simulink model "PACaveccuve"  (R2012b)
settings: Solver=ode45  StartTime=0.0  StopTime=6000  RelTol=1e-3
libraries: fl_lib x9, nesl_utility x6

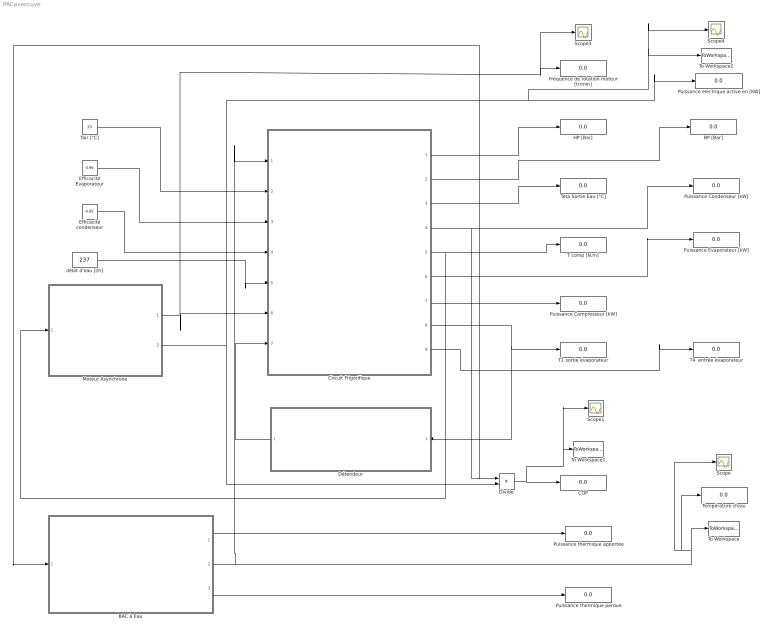
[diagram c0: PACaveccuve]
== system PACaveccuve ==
  BAC à Eau : Subsystem
  BP [Bar] : Display
  COP : Display
  Circuit Frigorifique : Subsystem
  Divide : Product  Inputs=*/
  Détendeur : Subsystem
  Efficacité Evaporateur : Constant  Value=0.99
  Efficacité condenseur : Constant  Value=0.95
  Fréquence de rotation moteur [tr/min] : Display
  HP [Bar] : Display
  Moteur Asynchrone : Subsystem
  Puissance Compresseur [kW] : Display
  Puissance Condenseur [kW] : Display
  Puissance Evaporateur [kW] : Display
  Puissance electrique active en [KW] : Display
  Puissance thermique apportée : Display
  Puissance thermique perdue : Display
  Scope{,1,3..4} (4 alike) : Scope
  T comp [N.m] : Display
  T1 sortie évaporateur : Display
  T4  entrée évaporateur : Display
  Tair [°C] : Constant  Value=23
  Température d'eau : Display
  Teta Sortie Eau [°C] : Display
  To Workspace : ToWorkspace  VariableName=Ts  SampleTime=-1  SaveFormat=Timeseries
  To Workspace1 : ToWorkspace  VariableName=COP  SampleTime=-1  SaveFormat=Timeseries
  To Workspace2 : ToWorkspace  VariableName=Pelec  SampleTime=-1  SaveFormat=Timeseries
  débit d'eau [l/h] : Constant  Value=237
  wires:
  Efficacité Evaporateur/1 -> Circuit Frigorifique/3(Eff Evapo)
  débit d'eau [l/h]/1 -> Circuit Frigorifique/5(Qv eau [l/h])
  Circuit Frigorifique/1(HP [bar]) -> HP [Bar]/1
  Circuit Frigorifique/2(BP [bar]) -> BP [Bar]/1
  Circuit Frigorifique/3(Tse [°C]) -> Teta Sortie Eau [°C]/1
  Circuit Frigorifique/5(Tm [N.m]) -> Moteur Asynchrone/1(Tm [N.m]), T comp [N.m]/1
  Circuit Frigorifique/9(T4 [°C]) -> T4  entrée évaporateur/1
  Circuit Frigorifique/8(T1 [°C]) -> Détendeur/1(T1), T1 sortie évaporateur/1
  Circuit Frigorifique/6(Pevapo [kW]) -> Puissance Evaporateur [kW]/1
  Divide/1 -> To Workspace1/1, Scope1/1, COP/1
  Circuit Frigorifique/7(Pcomp [kW]) -> Puissance Compresseur [kW]/1
  Efficacité condenseur/1 -> Circuit Frigorifique/4(effc)
  Détendeur/1(BP [Bar]) -> Circuit Frigorifique/7(BP[Bar])
  Moteur Asynchrone/2(Puissance Electrique active [W]) -> Scope4/1, To Workspace2/1, Puissance electrique active en [KW]/1, Divide/2
  Moteur Asynchrone/1(N [tr/min]) -> Scope3/1, Fréquence de rotation moteur [tr/min]/1, Circuit Frigorifique/6(N [tr/min])
  Tair [°C]/1 -> Circuit Frigorifique/2(Tair [°C])
  Circuit Frigorifique/4(Pcond [kW]) -> BAC à Eau/1(" Puissance Condenseur [kW]"), Divide/1, Puissance Condenseur [kW]/1
  BAC à Eau/2(Température du BAC [°C]) -> Scope/1, Température d'eau/1, To Workspace/1, Circuit Frigorifique/1(Tee [°C])
  BAC à Eau/1(Puissance Condenseur [W]) -> Puissance thermique apportée/1
  BAC à Eau/3(Puissance thermique perdue [W]) -> Puissance thermique perdue/1

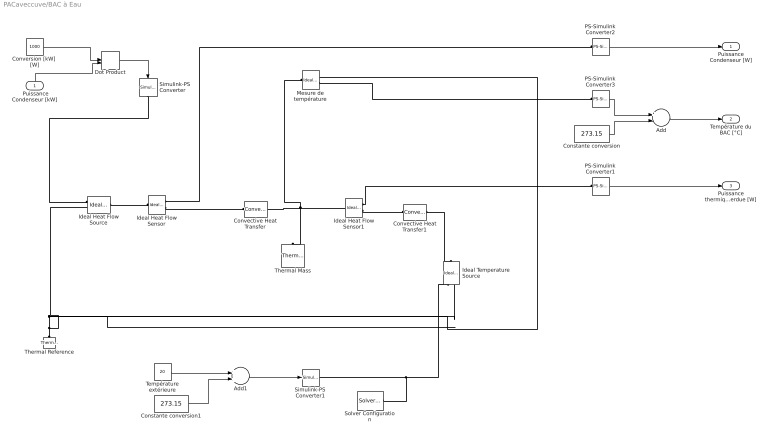
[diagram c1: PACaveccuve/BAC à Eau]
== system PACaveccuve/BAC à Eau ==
  " Puissance Condenseur [kW]" : Inport
  Add : Sum  Inputs=+-
  Add1 : Sum
  Constante conversion : Constant  Value=273.15
  Constante conversion1 : Constant  Value=273.15
  Convective Heat Transfer : fl_lib/Thermal/Thermal Elements/Convective Heat Transfer  area=1 m^2  heat_tr_coeff=1000000 W/(m^2 * K)  Q_Log=off  T_Log=off  LocalVarNames=|Q|T  LocalVarDescs=|Q|T  LocalVarLogging=[0 0]
  Convective Heat Transfer1 : fl_lib/Thermal/Thermal Elements/Convective Heat Transfer  area=1 m^2  heat_tr_coeff=10.3 W/(m^2 * K)  Q_Log=off  T_Log=off  LocalVarNames=|Q|T  LocalVarDescs=|Q|T  LocalVarLogging=[0 0]
  Conversion [kW]  [W] : Constant  Value=1000
  Dot Product : DotProduct
  Ideal Heat Flow Sensor : fl_lib/Thermal/Thermal Sensors/Ideal Heat Flow Sensor  Q_Log=off  T_Log=off  LocalVarNames=|Q|T  LocalVarDescs=|Q|T  LocalVarLogging=[0 0]
  Ideal Heat Flow Sensor1 : fl_lib/Thermal/Thermal Sensors/Ideal Heat Flow Sensor  Q_Log=off  T_Log=off  LocalVarNames=|Q|T  LocalVarDescs=|Q|T  LocalVarLogging=[0 0]
  Ideal Heat Flow Source : fl_lib/Thermal/Thermal Sources/Ideal Heat Flow Source  Q_Log=off  T_Log=off  LocalVarNames=|Q|T  LocalVarDescs=|Q|T  LocalVarLogging=[0 0]
  Ideal Temperature Source : fl_lib/Thermal/Thermal Sources/Ideal Temperature Source  Q_Log=off  T_Log=off  LocalVarNames=|Q|T  LocalVarDescs=|Q|T  LocalVarLogging=[0 0]
  Mesure de température : fl_lib/Thermal/Thermal Sensors/Ideal Temperature Sensor  Qs_Log=off  Ts_Log=off  LocalVarNames=|Qs|Ts  LocalVarDescs=|Qs|Ts  LocalVarLogging=[]
  PS-Simulink Converter1 : nesl_utility/PS-Simulink Converter  PhysicalDomain=network_engine_domain  LeftPortType=input  RightPortType=output  SubClassName=ps_output  PseudoPeriodic=off  Frequencies=[]  Unit=1  AffineConversion=off
  PS-Simulink Converter2 : nesl_utility/PS-Simulink Converter  PhysicalDomain=network_engine_domain  LeftPortType=input  RightPortType=output  SubClassName=ps_output  PseudoPeriodic=off  Frequencies=[]  Unit=1  AffineConversion=off
  PS-Simulink Converter3 : nesl_utility/PS-Simulink Converter  PhysicalDomain=network_engine_domain  LeftPortType=input  RightPortType=output  SubClassName=ps_output  PseudoPeriodic=off  Frequencies=[]  Unit=1  AffineConversion=off
  Simulink-PS Converter : nesl_utility/Simulink-PS Converter  PhysicalDomain=network_engine_domain  LeftPortType=input  RightPortType=output  SubClassName=ps_input  PseudoPeriodic=off  Frequencies=[]  NoiseDistribution=none  NoiseParameters=[]  Unit=1  AffineConversion=off  InputFilterTimeConstant=.001  UdotUserProvided=1  SimscapeFilterOrder=1  InputFiltering=off
  Simulink-PS Converter1 : nesl_utility/Simulink-PS Converter  PhysicalDomain=network_engine_domain  LeftPortType=input  RightPortType=output  SubClassName=ps_input  PseudoPeriodic=off  Frequencies=[]  NoiseDistribution=none  NoiseParameters=[]  Unit=K  AffineConversion=on  InputFilterTimeConstant=.001  UdotUserProvided=1  SimscapeFilterOrder=1  InputFiltering=off
  Solver Configuration : nesl_utility/Solver Configuration  PhysicalDomain=network_engine_domain  LeftPortType=input  RightPortType=generic  SubClassName=solver  Accelerate=off  Profile=off  UseLocalSampling=off  FrequencyDomain=off  Tones=[]  Harmonics=[]  UseCCode=off  SimulateNoise=off  EnableSwitchedLinearOptims=on  DoDC=off  ResidualTolerance=1e-9  UseLocalSolver=off  LocalSolverChoice=NE_BACKWARD_EULER_ADVANCER  LocalSolverSampleTime=.001  DoFixedCost=off  MaxNonlinIter=3  MaxModeIter=2  LinearAlgebra=Sparse  DelaysMemoryBudget=1024
  Température extérieure : Constant  Value=20
  Thermal Mass : fl_lib/Thermal/Thermal Elements/Thermal Mass  mass=19.9 kg  sp_heat=4185 J/kg/K  init_temp=23.25 C  Q_Log=off  LocalVarNames=|Q  LocalVarDescs=|Q  LocalVarLogging=0
  Thermal Reference : fl_lib/Thermal/Thermal Elements/Thermal Reference  Q_Log=off  LocalVarNames=|Q  LocalVarDescs=|Q  LocalVarLogging=0
  Puissance Condenseur [W] : Outport
  Température du BAC [°C] : Outport  Port=2
  Puissance thermique perdue [W] : Outport  Port=3
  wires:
  " Puissance Condenseur [kW]"/1 -> Dot Product/2
  PS-Simulink Converter3/1 -> Add/1
  Add/1 -> Température du BAC [°C]/1
  Constante conversion/1 -> Add/2
  Dot Product/1 -> Simulink-PS Converter/1
  Conversion [kW]  [W]/1 -> Dot Product/1
  PS-Simulink Converter1/1 -> Puissance thermique perdue [W]/1
  PS-Simulink Converter2/1 -> Puissance Condenseur [W]/1
  Add1/1 -> Simulink-PS Converter1/1
  Température extérieure/1 -> Add1/1
  Constante conversion1/1 -> Add1/2
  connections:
  Thermal Reference/LConn1 -- Ideal Temperature Source/RConn2 -- Mesure de température/RConn1 -- Ideal Heat Flow Source/RConn2
  Mesure de température/LConn1 -- Thermal Mass/LConn1 -- Ideal Heat Flow Sensor1/LConn1 -- Convective Heat Transfer/RConn1
  Solver Configuration/RConn1 -- Ideal Temperature Source/RConn1 -- Simulink-PS Converter1/RConn1
  Simulink-PS Converter/RConn1 -- Ideal Heat Flow Source/RConn1
  Convective Heat Transfer1/RConn1 -- Ideal Temperature Source/LConn1
  PS-Simulink Converter3/LConn1 -- Mesure de température/RConn2
  Ideal Heat Flow Source/LConn1 -- Ideal Heat Flow Sensor/LConn1
  Ideal Heat Flow Sensor/RConn2 -- Convective Heat Transfer/LConn1
  Ideal Heat Flow Sensor1/RConn2 -- Convective Heat Transfer1/LConn1
  Ideal Heat Flow Sensor1/RConn1 -- PS-Simulink Converter1/LConn1
  Ideal Heat Flow Sensor/RConn1 -- PS-Simulink Converter2/LConn1

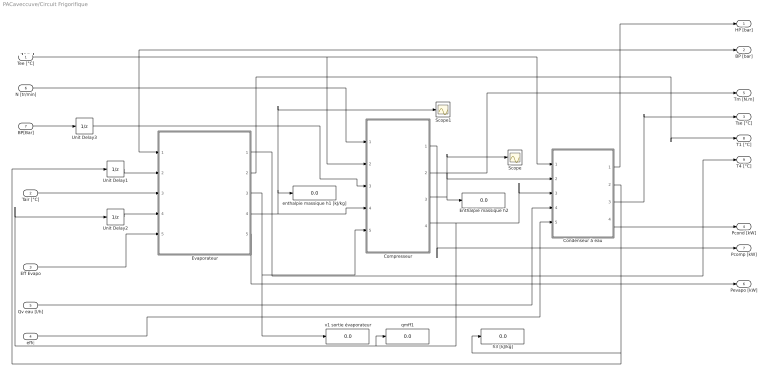
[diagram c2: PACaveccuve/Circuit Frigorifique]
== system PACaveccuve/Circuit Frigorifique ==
  note: +++++
  Tee [°C] : Inport
  Tair [°C] : Inport  Port=2
  Eff Evapo : Inport  Port=3
  effc : Inport  Port=4
  Qv eau [l/h] : Inport  Port=5
  N [tr/min] : Inport  Port=6
  BP[Bar] : Inport  Port=7
  Compresseur : Subsystem
  Condenseur à eau : Subsystem
  Enthalpie massique h2 : Display
  Evaporateur : Subsystem
  Scope : Scope
  Scope1 : Scope
  Unit Delay1 : UnitDelay  InitialCondition=300  SampleTime=-1
  Unit Delay2 : UnitDelay  InitialCondition=0.00001  SampleTime=-1
  Unit Delay3 : UnitDelay  InitialCondition=2.5  SampleTime=-1
  enthalpie massique h1 [kJ/kg] : Display
  h3 [kJ/kg] : Display
  qmff1 : Display
  v1 sortie évaporateur : Display
  HP [bar] : Outport
  BP [bar] : Outport  Port=2
  Tse [°C] : Outport  Port=3
  Pcond [kW] : Outport  Port=4
  Tm [N.m] : Outport  Port=5
  Pevapo [kW] : Outport  Port=6
  Pcomp [kW] : Outport  Port=7
  T1 [°C] : Outport  Port=8
  T4 [°C] : Outport  Port=9
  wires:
  Evaporateur/2(T1 [°C]) -> T1 [°C]/1
  N [tr/min]/1 -> Compresseur/1(N [tr/min])
  Evaporateur/5(Pévapo [kW]) -> Pevapo [kW]/1
  Tair [°C]/1 -> Evaporateur/3(Tair [°C])
  Condenseur à eau/3(Tse [°C]) -> Tse [°C]/1
  Unit Delay2/1 -> Evaporateur/4(qmff [kg/s])
  Condenseur à eau/1(HP [bar]) -> HP [bar]/1
  BP[Bar]/1 -> Unit Delay3/1
  Compresseur/4(qmff [kg/s]) -> Unit Delay2/1, qmff1/1, Condenseur à eau/3(qmff [kg/s])
  Tee [°C]/1 -> Compresseur/2(Tee [°C]), Condenseur à eau/1(Tee [°C])
  Eff Evapo/1 -> Evaporateur/5(Eff)
  Qv eau [l/h]/1 -> Condenseur à eau/4(qveau [l/h])
  Evaporateur/3(v1 [m3/kg]) -> v1 sortie évaporateur/1, Compresseur/5(v1 [m3/kg])
  Condenseur à eau/2(h3 [kJ/kg]) -> Unit Delay1/1, h3 [kJ/kg]/1
  Evaporateur/4(h1 [kJ/kg]) -> Compresseur/4(h1 [kJ/kg]), Scope1/1, enthalpie massique h1 [kJ/kg]/1
  Compresseur/3(h2 [kJ/kg]) -> Scope/1, Condenseur à eau/2(h2 [kJ/kg]), Enthalpie massique h2/1
  Compresseur/2(Tm [N.m]) -> Tm [N.m]/1
  Evaporateur/1(T4 [°C]) -> T4 [°C]/1
  Condenseur à eau/4(Pcond [kW]) -> Pcond [kW]/1
  Unit Delay1/1 -> Evaporateur/2(h3 [kJ/kg])
  Compresseur/1(Pcomp [kW]) -> Pcomp [kW]/1
  effc/1 -> Condenseur à eau/5(effc)
  Unit Delay3/1 -> BP [bar]/1, Compresseur/3(BP [bar]), Evaporateur/1(BP [bar])

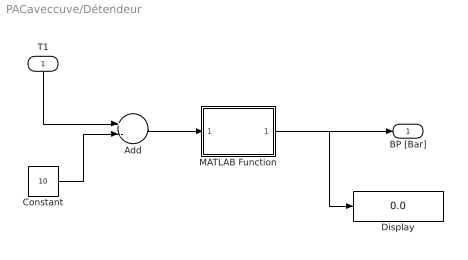
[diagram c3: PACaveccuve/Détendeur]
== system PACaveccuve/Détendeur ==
  T1 : Inport
  Add : Sum  Inputs=+-
  Constant : Constant  Value=10
  Display : Display
  MATLAB Function : MATLAB Function  TreatAsAtomicUnit=on
  BP [Bar] : Outport
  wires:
  Add/1 -> MATLAB Function/1(T)
  T1/1 -> Add/1
  Constant/1 -> Add/2
  MATLAB Function/1(BP) -> Display/1, BP [Bar]/1

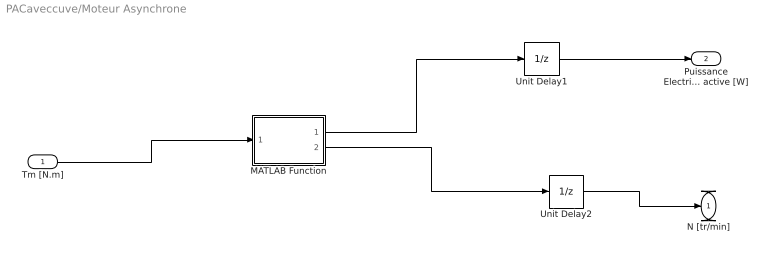
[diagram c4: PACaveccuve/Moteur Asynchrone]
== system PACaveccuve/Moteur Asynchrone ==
  Tm [N.m] : Inport
  MATLAB Function : MATLAB Function  TreatAsAtomicUnit=on
  Unit Delay1 : UnitDelay  InitialCondition=0.2  SampleTime=-1
  Unit Delay2 : UnitDelay  InitialCondition=1480  SampleTime=-1
  N [tr/min] : Outport
  Puissance Electrique active [W] : Outport  Port=2
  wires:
  Unit Delay1/1 -> Puissance Electrique active [W]/1
  Unit Delay2/1 -> N [tr/min]/1
  Tm [N.m]/1 -> MATLAB Function/1(Tm)
  MATLAB Function/1(P) -> Unit Delay1/1
  MATLAB Function/2(N) -> Unit Delay2/1

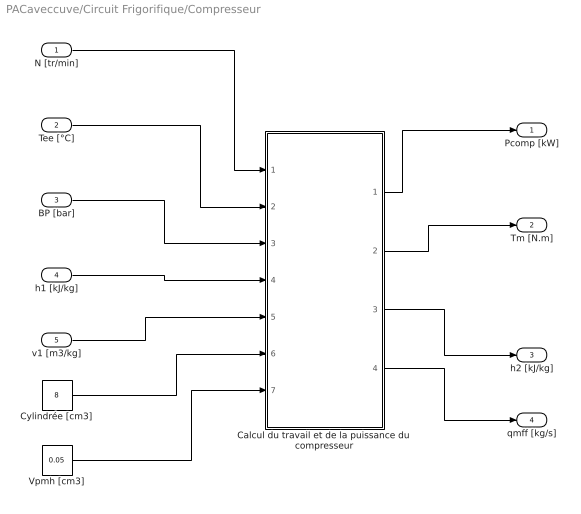
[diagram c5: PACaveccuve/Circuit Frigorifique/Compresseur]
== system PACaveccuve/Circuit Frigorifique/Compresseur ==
  N [tr/min] : Inport
  Tee [°C] : Inport  Port=2
  BP [bar] : Inport  Port=3
  h1 [kJ/kg] : Inport  Port=4
  v1 [m3/kg] : Inport  Port=5
  Calcul du travail et de la puissance du compresseur : MATLAB Function  TreatAsAtomicUnit=on
  Cylindrée [cm3] : Constant  Value=8
  Vpmh [cm3] : Constant  Value=0.05
  Pcomp [kW] : Outport
  Tm [N.m] : Outport  Port=2
  h2 [kJ/kg] : Outport  Port=3
  qmff [kg/s] : Outport  Port=4
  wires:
  Calcul du travail et de la puissance du compresseur/4(qmff) -> qmff [kg/s]/1
  Calcul du travail et de la puissance du compresseur/2(Tm) -> Tm [N.m]/1
  h1 [kJ/kg]/1 -> Calcul du travail et de la puissance du compresseur/4(h1)
  Tee [°C]/1 -> Calcul du travail et de la puissance du compresseur/2(Tee)
  BP [bar]/1 -> Calcul du travail et de la puissance du compresseur/3(BP)
  Calcul du travail et de la puissance du compresseur/1(P) -> Pcomp [kW]/1
  Calcul du travail et de la puissance du compresseur/3(h2) -> h2 [kJ/kg]/1
  N [tr/min]/1 -> Calcul du travail et de la puissance du compresseur/1(N)
  v1 [m3/kg]/1 -> Calcul du travail et de la puissance du compresseur/5(v1)
  Cylindrée [cm3]/1 -> Calcul du travail et de la puissance du compresseur/6(cyl)
  Vpmh [cm3]/1 -> Calcul du travail et de la puissance du compresseur/7(Vpmh)

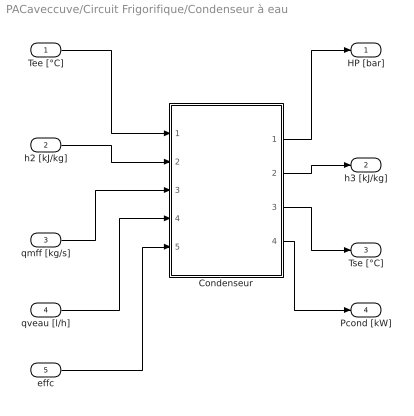
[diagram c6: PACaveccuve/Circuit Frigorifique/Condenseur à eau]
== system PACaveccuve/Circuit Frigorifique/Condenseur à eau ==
  Tee [°C] : Inport
  h2 [kJ/kg] : Inport  Port=2
  qmff [kg/s] : Inport  Port=3
  qveau [l/h] : Inport  Port=4
  effc : Inport  Port=5
  Condenseur : MATLAB Function  TreatAsAtomicUnit=on
  HP [bar] : Outport
  h3 [kJ/kg] : Outport  Port=2
  Tse [°C] : Outport  Port=3
  Pcond [kW] : Outport  Port=4
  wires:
  Tee [°C]/1 -> Condenseur/1(Tee)
  Condenseur/3(Tse) -> Tse [°C]/1
  Condenseur/1(HP) -> HP [bar]/1
  h2 [kJ/kg]/1 -> Condenseur/2(h2)
  qmff [kg/s]/1 -> Condenseur/3(qmff)
  qveau [l/h]/1 -> Condenseur/4(qveau)
  Condenseur/2(h3) -> h3 [kJ/kg]/1
  Condenseur/4(Pcond) -> Pcond [kW]/1
  effc/1 -> Condenseur/5(eff)

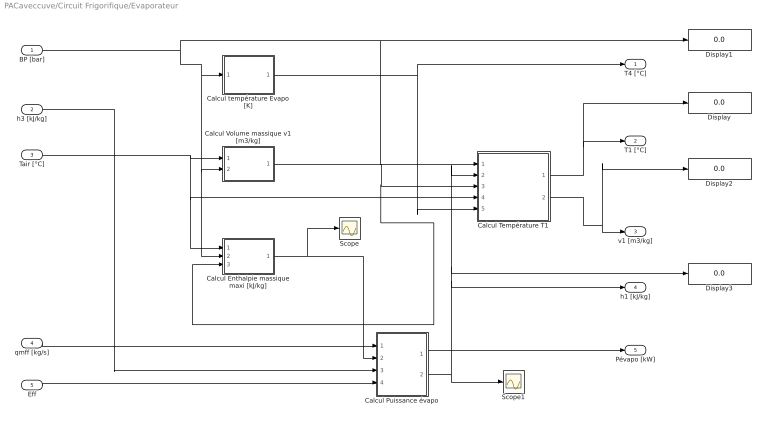
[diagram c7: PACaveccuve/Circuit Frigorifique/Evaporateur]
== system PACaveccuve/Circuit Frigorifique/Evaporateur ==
  BP [bar] : Inport
  h3 [kJ/kg] : Inport  Port=2
  Tair [°C] : Inport  Port=3
  qmff [kg/s] : Inport  Port=4
  Eff : Inport  Port=5
  Calcul Enthalpie massique maxi [kJ/kg] : MATLAB Function  TreatAsAtomicUnit=on
  Calcul Puissance évapo : MATLAB Function  TreatAsAtomicUnit=on
  Calcul Température T1 : MATLAB Function  TreatAsAtomicUnit=on
  Calcul Volume massique v1 [m3/kg] : MATLAB Function  TreatAsAtomicUnit=on
  Calcul température Evapo [K] : MATLAB Function  TreatAsAtomicUnit=on
  Display{,1..3} (4 alike) : Display
  Scope : Scope
  Scope1 : Scope
  T4 [°C] : Outport
  T1 [°C] : Outport  Port=2
  v1 [m3/kg] : Outport  Port=3
  h1 [kJ/kg] : Outport  Port=4
  Pévapo [kW] : Outport  Port=5
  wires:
  qmff [kg/s]/1 -> Calcul Puissance évapo/1(qmff)
  Calcul Enthalpie massique maxi [kJ/kg]/1(H) -> Scope/1, Calcul Puissance évapo/2(hmax)
  BP [bar]/1 -> Calcul Enthalpie massique maxi [kJ/kg]/2(P), Calcul Volume massique v1 [m3/kg]/2(P), Calcul température Evapo [K]/1(P), Display1/1, Calcul Température T1/1(P)
  Calcul température Evapo [K]/1(T) -> T4 [°C]/1, Calcul Température T1/5(T3)
  Tair [°C]/1 -> Calcul Enthalpie massique maxi [kJ/kg]/1(T), Calcul Température T1/4(T1max), Calcul Volume massique v1 [m3/kg]/1(T)
  Calcul Puissance évapo/1(Pevapo) -> Pévapo [kW]/1
  Eff/1 -> Calcul Puissance évapo/4(eff)
  Calcul Volume massique v1 [m3/kg]/1(v) -> Calcul Enthalpie massique maxi [kJ/kg]/3(v), Calcul Température T1/3(v)
  Calcul Température T1/2(v1) -> Display2/1, v1 [m3/kg]/1
  Calcul Température T1/1(T1) -> Display/1, T1 [°C]/1
  Calcul Puissance évapo/2(h1) -> h1 [kJ/kg]/1, Display3/1, Calcul Température T1/2(h), Scope1/1
  h3 [kJ/kg]/1 -> Calcul Puissance évapo/3(h3)
